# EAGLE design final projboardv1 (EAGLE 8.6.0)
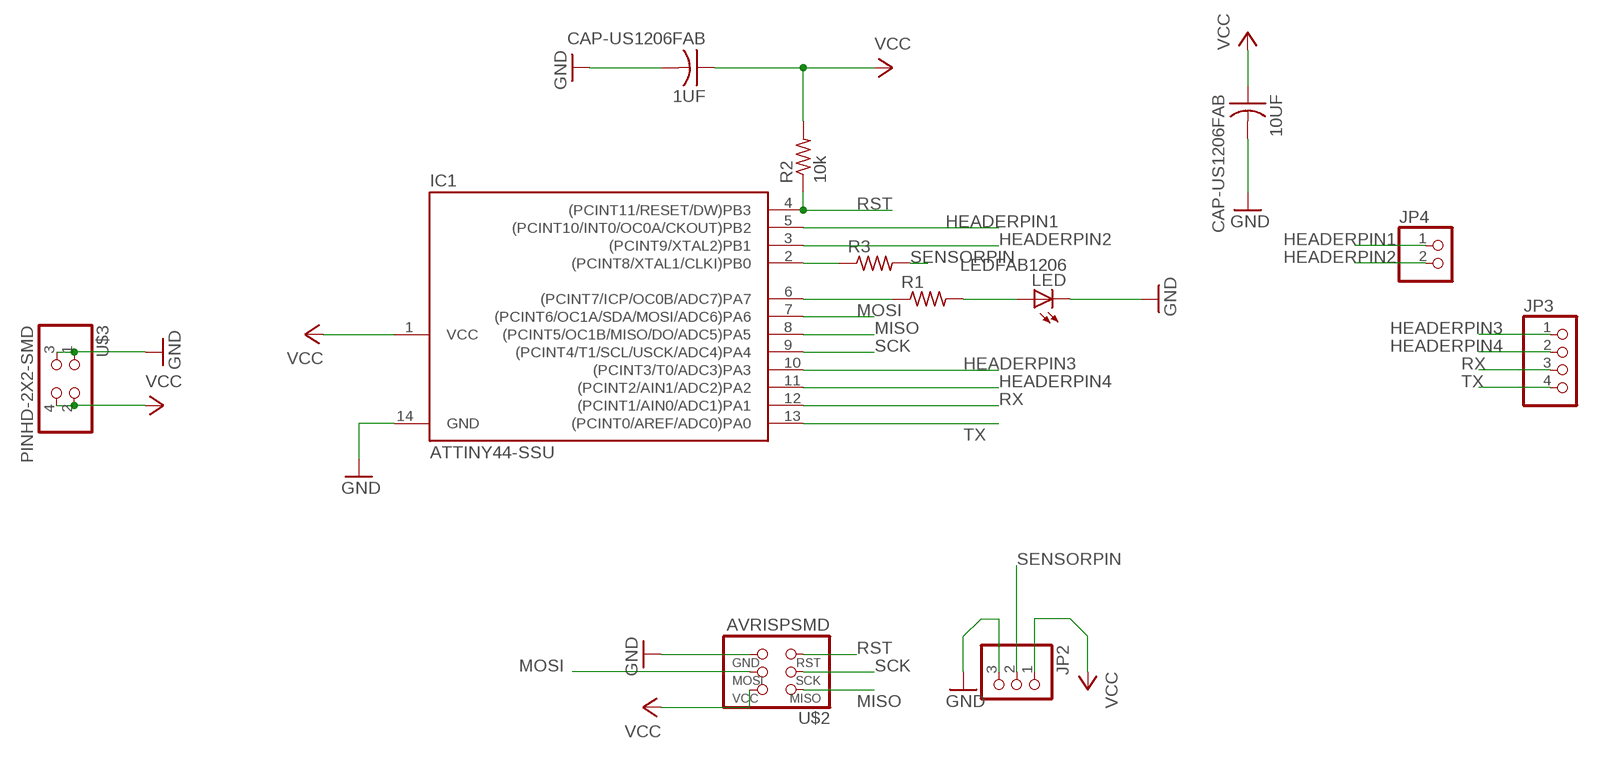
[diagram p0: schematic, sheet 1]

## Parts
1UF  CAP-US1206FAB  [C1206FAB]
10UF  CAP-US1206FAB  [C1206FAB]
IC1  ATTINY44-SSU  [SOIC14]
JP2  PINHD-1X3  [1X03]
JP3  PINHD-1X4  [1X04]
JP4  PINHD-1X2  [1X02]
LED  LEDFAB1206  [LED1206FAB]
R1  RES-US1206FAB  [R1206FAB]
R2  10k  RES-US1206FAB  [R1206FAB]
R3  RES-US1206FAB  [R1206FAB]
U$2  AVRISPSMD  [2X03SMD]
U$3  PINHD-2X2-SMD  [2X02SMD]

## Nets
GND: 1UF.2 10UF.2 IC1.14(GND) JP2.3 LED.2(C) U$2.6(GND) U$3.1 U$3.3
HEADERPIN1: IC1.5((PCINT10/INT0/OC0A/CKOUT)PB2) JP4.1
HEADERPIN2: IC1.3((PCINT9/XTAL2)PB1) JP4.2
HEADERPIN3: IC1.10((PCINT3/T0/ADC3)PA3) JP3.1
HEADERPIN4: IC1.11((PCINT2/AIN1/ADC2)PA2) JP3.2
MISO: IC1.8((PCINT5/OC1B/MISO/DO/ADC5)PA5) U$2.1(MISO)
MOSI: IC1.7((PCINT6/OC1A/SDA/MOSI/ADC6)PA6) U$2.4(MOSI)
N$1: IC1.2((PCINT8/XTAL1/CLKI)PB0) R3.1
N$3: IC1.6((PCINT7/ICP/OC0B/ADC7)PA7) R1.1
N$4: LED.1(A) R1.2
RST: IC1.4((PCINT11/RESET/DW)PB3) R2.1 U$2.5(RST)
RX: IC1.12((PCINT1/AIN0/ADC1)PA1) JP3.3
SCK: IC1.9((PCINT4/T1/SCL/USCK/ADC4)PA4) U$2.3(SCK)
SENSORPIN: JP2.2 R3.2
TX: IC1.13((PCINT0/AREF/ADC0)PA0) JP3.4
VCC: 1UF.1 10UF.1 IC1.1(VCC) JP2.1 R2.2 U$2.2(VCC) U$3.2 U$3.4

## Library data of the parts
1UF 10UF = fab:CAP-US
IC1 = fab:ATTINY44
JP2 = pinhead:PINHD-1X3: PIN HEADER
JP3 = pinhead:PINHD-1X4: PIN HEADER
JP4 = pinhead:PINHD-1X2: PIN HEADER
LED = fab:LED: LED
R1-R3 = fab:RES-US: Resistor (US Symbol)
U$2 = fab:AVRISP
U$3 = fab:PINHD-2X2-SMD

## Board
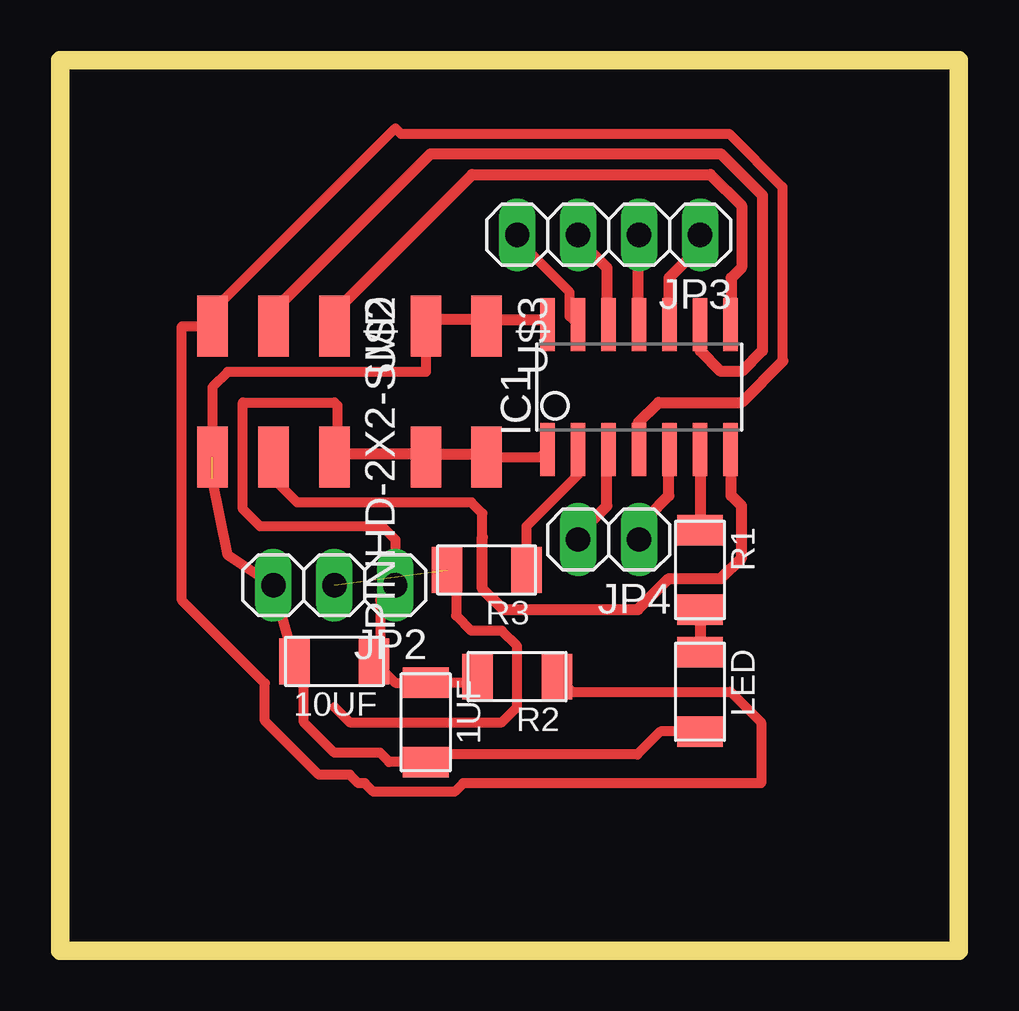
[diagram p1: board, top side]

Size 37.45 x 37.14 mm. Coordinates in mm from the lower left corner, seen from the top.
Outline: 0,0 37.45,0 37.45,37.14 0,37.14 0,0
Copper layers (1*16): Top 0.035mm / dielectric 1.5mm / Bottom 0.035mm
Design rules "default *": minimum track width 18mil, minimum drill 0.35mm, track to track 16mil, track to pad 16mil, pad to pad 16mil, via to via 16mil, smd to smd 16mil, copper to edge 40mil, drill to drill 16mil, minimum pad ring 10mil, minimum via ring 8mil, stop-mask expansion 4mil, vias tented up to drill 0mil, thermal gap 10mil

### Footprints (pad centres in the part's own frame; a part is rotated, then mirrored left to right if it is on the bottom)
C1206FAB = smd 1.27 x 1.905: 1 -1.651,0; 2 1.651,0
SOIC14 = smd 0.61 x 2.21: 1 -3.81,-2.603; 2 -2.54,-2.603; 3 -1.27,-2.603; 4 0,-2.603; 5 1.27,-2.603; 6 2.54,-2.603; 7 3.81,-2.603; 8 3.81,2.603; 9 2.54,2.603; 10 1.27,2.603; 11 0,2.603; 12 -1.27,2.603; 13 -2.54,2.603; 14 -3.81,2.603
1X03 = drill 1.016 long: 1 -2.54,0; 2 0,0; 3 2.54,0
1X04 = drill 1.016 long: 1 -3.81,0; 2 -1.27,0; 3 1.27,0; 4 3.81,0
1X02 = drill 1.016 long: 1 -1.27,0; 2 1.27,0
LED1206FAB = smd 1.27 x 1.905: 1 -1.651,0; 2 1.651,0
R1206FAB = smd 1.27 x 1.905: 1 -1.651,0; 2 1.651,0
2X03SMD = smd 2.54 x 1.27: 1 -2.54,2.54; 2 2.92,2.54; 3 -2.54,0; 4 2.92,0; 5 -2.54,-2.54; 6 2.92,-2.54
2X02SMD = smd 2.54 x 1.27: 1 -2.54,1.27; 2 2.92,1.27; 3 -2.54,-1.27; 4 2.92,-1.27

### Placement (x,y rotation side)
1UF  15.24,9.53 270 top
10UF  11.43,12.07 180 top
IC1  24.13,23.5 0 top
JP2  11.43,15.24 180 top
JP3  22.86,29.85 180 top
JP4  22.86,17.14 180 top
LED  26.67,10.79 270 top
R1  26.67,15.88 270 top
R2  19.05,11.43 180 top
R3  17.78,15.88 180 top
U$2  8.89,23.5 270 top
U$3  16.51,23.5 270 top

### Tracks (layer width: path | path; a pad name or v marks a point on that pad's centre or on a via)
GND  (1 unrouted)
  Top 0.406: 14.86,8.25 1UF.2 13.72,7.87 13.34,8.25 11.43,8.25 10.16,9.53 10.16,11.68 10UF.2 JP2.3 6.98,16.51 6.35,19.68 | 15.44,8.18 24.05,8.18 25.02,9.14 LED.2 | U$3.3 15.24,24.13 6.98,24.13 6.35,23.5 U$2.6
  Top 0.457: IC1.14 20.19,26.31 18.03,26.31 U$3.1 17.6,26.31 15.44,26.31 U$3.3 | 26.67,9.04 LED.2 | 1UF.2 15.44,8.18
HEADERPIN1
  Top 0.457: IC1.5 25.38,20.7 25.38,18.97 24.51,18.11 24.51,17.25 JP4.1
HEADERPIN2
  Top 0.457: IC1.3 22.78,20.7 22.78,18.54 21.49,17.25 JP4.2
HEADERPIN3
  Top 0.457: JP3.1 26.67,29.34 25.38,28.04 25.38,26.31 IC1.10
HEADERPIN4
  Top 0.457: IC1.11 24.08,26.31 24.08,29.77 JP3.2
MISO
  Top 0.457: IC1.8 27.97,26.31 27.97,28.04 28.4,28.47 28.4,31.06 27.1,32.36 17.17,32.36 11.12,26.31 U$2.1
MOSI
  Top 0.406: 17.6,17.25 17.6,18.24 17.14,18.7 9.88,18.7 8.89,19.68 U$2.4
  Top 0.457: 17.6,17.25 17.6,15.09 18.47,14.22 24.08,14.22 25.38,15.52 27.53,15.52 28.4,16.38 28.4,18.54 27.97,18.97 27.97,20.7 IC1.7 | 8.53,20.27 U$2.4
N$1
  Top 0.406: R3.1 19.43,17.69 21.59,19.85 IC1.2
  Top 0.457: 19.33,15.95 R3.1
N$3
  Top 0.457: IC1.6 R1.1
N$4
  Top 0.457: R1.2 LED.1
RST
  Top 0.406: 30.12,24.59 30.1,24.61 30.1,31.84 27.88,34.06 14.2,34.06 13.97,34.29 6.35,26.67 U$2.5 5.08,26.04 5.08,14.61 8.53,11.15 8.53,9.59 10.78,7.34 12.07,7.34 12.43,6.99 12.7,6.99 13.06,6.63 16.45,6.63 16.8,6.99 29.21,6.99 29.21,9.53 27.94,10.79 21.34,10.79 R2.1
  Top 0.457: IC1.4 24.08,21.13 24.08,22 24.94,22.86 28.4,22.86 30.12,24.59 | 6.38,26.31 U$2.5
RX
  Top 0.457: IC1.12 22.78,26.31 22.78,28.47 21.49,29.77 JP3.3
SCK
  Top 0.457: IC1.9 26.67,25.02 27.53,24.16 28.4,24.16 29.26,25.02 29.26,31.5 27.53,33.22 15.44,33.22 8.53,26.31 U$2.3
SENSORPIN  (1 unrouted)
  Top 0.406: 11.43,10.16 12.06,9.53 18.42,9.53 19.05,10.16 19.05,12.7 18.42,13.34 17.14,13.34 16.51,13.97 16.51,15.49 R3.2
TX
  Top 0.406: IC1.13 21.23,26.45 21.23,27.46 19.05,29.64 JP3.4
VCC
  Top 0.406: U$3.2 20,20.57 IC1.1 | 10UF.1 13.21,11.94 | 13.21,11.94 13.97,11.18 1UF.1 17.14,11.18 R2.2 | 13.21,11.94 13.34,12.07 13.34,14.61 JP2.1 13.97,17.14 13.41,17.7 8.33,17.7 7.62,18.42 7.62,22.86 11.43,22.86 11.56,22.73 11.56,20.7
  Top 0.457: 15.44,11.2 1UF.1 | U$2.2 11.56,20.7 15.01,20.7 U$3.4 15.44,20.7 17.6,20.7 U$3.2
